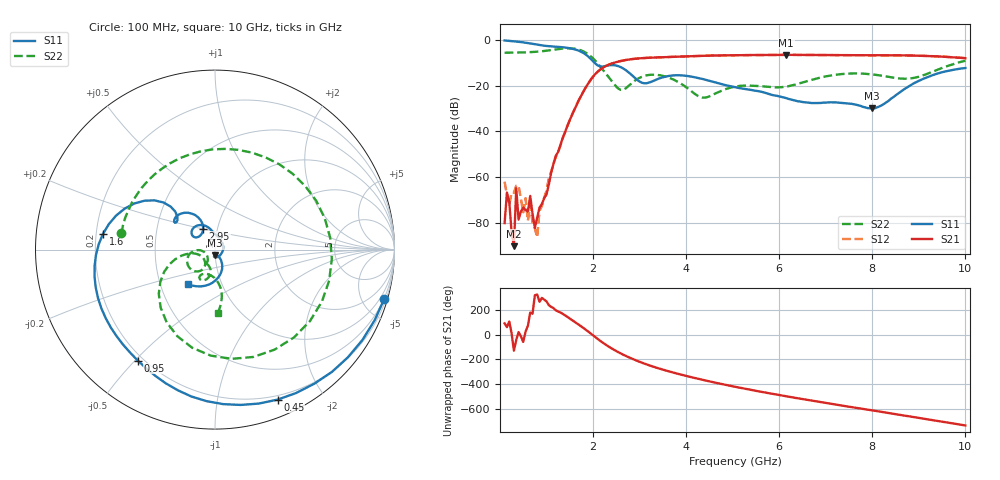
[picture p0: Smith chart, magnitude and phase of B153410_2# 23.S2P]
!  2-Port S-parameters saved by WinCal
! VAR MeasName=S-Parameters (CALIBRATED_DATA) read from VNA (N5245A)
! VAR MeasDate=2016-12-23 10:00:30
! VAR NAME=B153410_2# 23
! VAR FILENAME=B153410_2# 23.S2P
! VAR DATE=2016-12-23 10:00:30
! VAR PHYS_PORTS=1,2
# Hz S DB R 50
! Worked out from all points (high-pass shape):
!   199 points, 100 MHz to 10 GHz, reference 50 ohm
!   highest |S21| = -6.46 dB at 6.15 GHz (marker M1); lowest = -90.2 dB at 300 MHz (marker M2)
!   |S21| within 3 dB of the highest: 2.533 GHz to end of sweep
!   lowest |S11| = -29.9 dB at 8 GHz (marker M3), VSWR 1.07, Z = 50 - j3.21 ohm
!   |S11| at or under -10 dB: 2.037 GHz to end of sweep
!   |S22| runs from -25.2 to -3.6 dB; largest |S21 - S12| = 0.0026
!   S11 on the Smith chart (normalised r, x): 100 MHz: 0.45, -7.01; 450 MHz: 0.16, -1.49; 950 MHz: 0.18, -0.51; 1.6 GHz: 0.23, +0.07; 2.95 GHz: 0.85, +0.20; 10 GHz: 0.69, -0.28
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1e8  -0.15 -16.2  -80.10 94.1  -61.99 -75.0  -5.53 170.2
1.5e8  -0.24 -24.0  -66.72 63.4  -67.87 -129.8  -5.51 165.3
3e8  -0.51 -46.3  -90.21 -128.6  -66.84 -40.1  -5.48 150.3
3.5e8  -0.63 -53.4  -64.92 -40.9  -63.74 129.7  -5.48 145.0
4e8  -0.74 -60.5  -78.55 23.2  -63.70 69.0  -5.45 139.9
4.5e8  -0.86 -67.3  -75.06 -11.6  -69.43 102.5  -5.42 134.3
6e8  -1.29 -87.0  -74.93 74.2  -79.04 -56.7  -5.32 117.2
6.5e8  -1.46 -93.2  -68.21 -178.2  -72.22 65.0  -5.27 111.1
8e8  -2.00 -110.1  -77.67 -31.2  -86.31 29.0  -5.06 91.5
9.5e8  -2.46 -124.8  -69.24 -72.6  -68.95 -103.2  -4.76 69.4
1.3e9  -3.03 -157.5  -45.76 -177.6  -46.28 -177.0  -3.81 5.9
1.6e9  -4.01 172.0  -30.42 108.5  -30.38 108.9  -3.76 -59.2
1.75e9  -5.15 155.6  -24.13 68.4  -24.13 68.3  -4.57 -92.3
2.4e9  -10.93 141.0  -10.26 -110.3  -10.27 -110.5  -17.91 -170.6
2.95e9  -17.44 119.4  -8.07 148.3  -8.07 148.3  -17.04 -123.8
3.4e9  -16.96 148.8  -7.57 88.5  -7.57 88.4  -15.29 -153.2
5.05e9  -20.63 95.2  -6.59 -62.5  -6.62 -62.4  -20.37 -123.6
6.15e9  -25.41 37.3  -6.46 -139.8  -6.48 -139.8  -20.34 -111.5
6.7e9  -27.55 -26.8  -6.48 -175.5  -6.51 -175.4  -17.40 -100.9
8e9  -29.87 -87.8  -6.64 105.3  -6.63 105.2  -15.02 -119.6
8.35e9  -26.55 -62.7  -6.67 84.0  -6.65 84.2  -16.08 -117.9
1e10  -12.22 -128.6  -7.92 -17.4  -7.90 -17.4  -9.03 -87.7
